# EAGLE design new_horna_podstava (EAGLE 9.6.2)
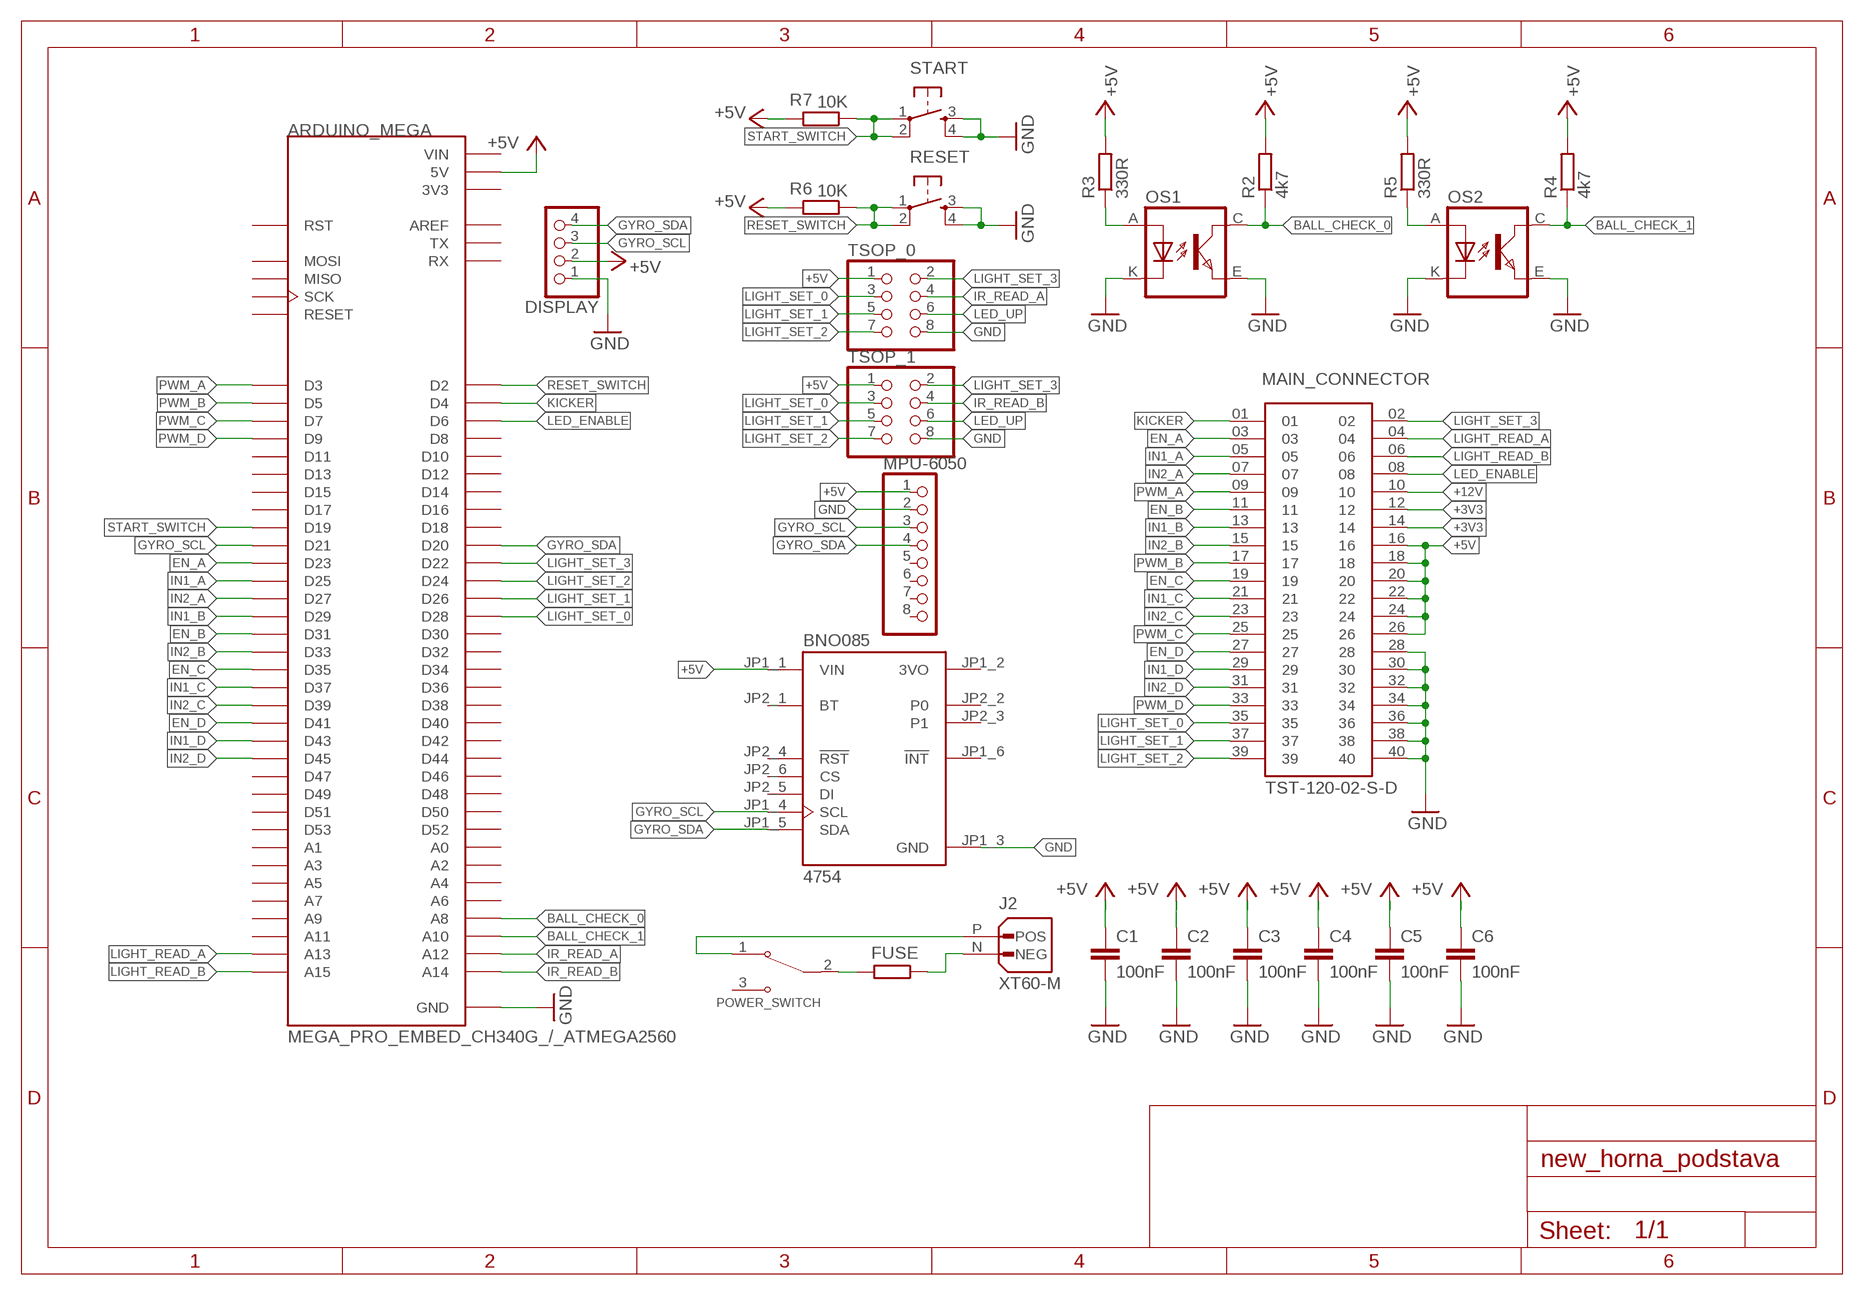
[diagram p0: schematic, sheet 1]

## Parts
ARDUINO_MEGA  MEGA_PRO_EMBED_CH340G_/_ATMEGA2560  [MODULE_MEGA_PRO_EMBED_CH340G_/_ATMEGA2560]
BNO085  4754  [MODULE_4754]
C1  100nF  C-EUC0805  [C0805]
C2  100nF  C-EUC0805  [C0805]
C3  100nF  C-EUC0805  [C0805]
C4  100nF  C-EUC0805  [C0805]
C5  100nF  C-EUC0805  [C0805]
C6  100nF  C-EUC0805  [C0805]
DISPLAY  PINHD-1X4  [1X04]
FUSE  R-EU_R1206  [R1206]
J2  XT60-M  [AMASS_XT60-M]
MAIN_CONNECTOR  TST-120-02-S-D  [SAMTEC_TST-120-02-S-D]
MPU-6050  PINHD-1X8  [1X08]
OS1  TCRT5000  [TCRT5000]
OS2  TCRT5000  [TCRT5000]
POWER_SWITCH  100SP1T1B4M2QE  [SW_100SP1T1B4M2QE]
R2  4k7  R-EU_R1206  [R1206]
R3  330R  R-EU_R1206  [R1206]
R4  4k7  R-EU_R1206  [R1206]
R5  330R  R-EU_R1206  [R1206]
R6  10K  R-EU_R1206  [R1206]
R7  10K  R-EU_R1206  [R1206]
RESET  DTSM-6  [DTSM-6]
START  DTSM-6  [DTSM-6]
TSOP_0  PINHD-2X4  [2X04]
TSOP_1  PINHD-2X4  [2X04]

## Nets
+3V3: MAIN_CONNECTOR.12 MAIN_CONNECTOR.14
+5V: ARDUINO_MEGA.5V_1(5V) ARDUINO_MEGA.5V_2(5V) ARDUINO_MEGA.5V_3(5V) BNO085.JP1_1(VIN) C1.1 C2.1 C3.1 C4.1 C5.1 C6.1 DISPLAY.2 MAIN_CONNECTOR.16 MAIN_CONNECTOR.18 MAIN_CONNECTOR.20 MAIN_CONNECTOR.22 MAIN_CONNECTOR.24 MAIN_CONNECTOR.26 MPU-6050.1 R2.2 R3.2 R4.2 R5.2 R6.2 R7.2 TSOP_0.1 TSOP_1.1
+12V: MAIN_CONNECTOR.10
BALL_CHECK_0: ARDUINO_MEGA.A8 OS1.C(COLLECTOR) R2.1
BALL_CHECK_1: ARDUINO_MEGA.A10 OS2.C(COLLECTOR) R4.1
EN_A: ARDUINO_MEGA.D23 MAIN_CONNECTOR.03
EN_B: ARDUINO_MEGA.D31 MAIN_CONNECTOR.11
EN_C: ARDUINO_MEGA.D35 MAIN_CONNECTOR.19
EN_D: ARDUINO_MEGA.D41 MAIN_CONNECTOR.27
GND: ARDUINO_MEGA.GND_1(GND) ARDUINO_MEGA.GND_2(GND) ARDUINO_MEGA.GND_3(GND) BNO085.JP1_3(GND) C1.2 C2.2 C3.2 C4.2 C5.2 C6.2 DISPLAY.1 MAIN_CONNECTOR.28 MAIN_CONNECTOR.30 MAIN_CONNECTOR.32 MAIN_CONNECTOR.34 MAIN_CONNECTOR.36 MAIN_CONNECTOR.38 MAIN_CONNECTOR.40 MPU-6050.2 OS1.E(EMITTER) OS1.K(CATHODE) OS2.E(EMITTER) OS2.K(CATHODE) RESET.3 RESET.4 START.3 START.4 TSOP_0.8 TSOP_1.8
GYRO_SCL: ARDUINO_MEGA.D21 BNO085.JP1_4(SCL) DISPLAY.3 MPU-6050.3
GYRO_SDA: ARDUINO_MEGA.D20 BNO085.JP1_5(SDA) DISPLAY.4 MPU-6050.4
IN1_A: ARDUINO_MEGA.D25 MAIN_CONNECTOR.05
IN1_B: ARDUINO_MEGA.D29 MAIN_CONNECTOR.13
IN1_C: ARDUINO_MEGA.D37 MAIN_CONNECTOR.21
IN1_D: ARDUINO_MEGA.D43 MAIN_CONNECTOR.29
IN2_A: ARDUINO_MEGA.D27 MAIN_CONNECTOR.07
IN2_B: ARDUINO_MEGA.D33 MAIN_CONNECTOR.15
IN2_C: ARDUINO_MEGA.D39 MAIN_CONNECTOR.23
IN2_D: ARDUINO_MEGA.D45 MAIN_CONNECTOR.31
IR_READ_A: ARDUINO_MEGA.A12 TSOP_0.4
IR_READ_B: ARDUINO_MEGA.A14 TSOP_1.4
KICKER: ARDUINO_MEGA.D4 MAIN_CONNECTOR.01
LED_ENABLE: ARDUINO_MEGA.D6 MAIN_CONNECTOR.08
LED_UP: TSOP_0.6 TSOP_1.6
LIGHT_READ_A: ARDUINO_MEGA.A13 MAIN_CONNECTOR.04
LIGHT_READ_B: ARDUINO_MEGA.A15 MAIN_CONNECTOR.06
LIGHT_SET_0: ARDUINO_MEGA.D28 MAIN_CONNECTOR.35 TSOP_0.3 TSOP_1.3
LIGHT_SET_1: ARDUINO_MEGA.D26 MAIN_CONNECTOR.37 TSOP_0.5 TSOP_1.5
LIGHT_SET_2: ARDUINO_MEGA.D24 MAIN_CONNECTOR.39 TSOP_0.7 TSOP_1.7
LIGHT_SET_3: ARDUINO_MEGA.D22 MAIN_CONNECTOR.02 TSOP_0.2 TSOP_1.2
N$1: FUSE.2 POWER_SWITCH.2
N$2: J2.P(POS) POWER_SWITCH.1
N$3: FUSE.1 J2.N(NEG)
N$5: OS2.A(ANODE) R5.1
N$6: OS1.A(ANODE) R3.1
PWM_A: ARDUINO_MEGA.D3 MAIN_CONNECTOR.09
PWM_B: ARDUINO_MEGA.D5 MAIN_CONNECTOR.17
PWM_C: ARDUINO_MEGA.D7 MAIN_CONNECTOR.25
PWM_D: ARDUINO_MEGA.D9 MAIN_CONNECTOR.33
RESET_SWITCH: ARDUINO_MEGA.D2 R6.1 RESET.1 RESET.2
START_SWITCH: ARDUINO_MEGA.D19 R7.1 START.1 START.2
Unconnected: ARDUINO_MEGA.A0 ARDUINO_MEGA.A1 ARDUINO_MEGA.A2 ARDUINO_MEGA.A3 ARDUINO_MEGA.A4 ARDUINO_MEGA.A5 ARDUINO_MEGA.A6 ARDUINO_MEGA.A7 ARDUINO_MEGA.A9 ARDUINO_MEGA.A11 ARDUINO_MEGA.AREF ARDUINO_MEGA.D8 ARDUINO_MEGA.D10 ARDUINO_MEGA.D11 ARDUINO_MEGA.D12 ARDUINO_MEGA.D13 ARDUINO_MEGA.D14 ARDUINO_MEGA.D15 ARDUINO_MEGA.D16 ARDUINO_MEGA.D17 ARDUINO_MEGA.D18 ARDUINO_MEGA.D30 ARDUINO_MEGA.D32 ARDUINO_MEGA.D34 ARDUINO_MEGA.D36 ARDUINO_MEGA.D38 ARDUINO_MEGA.D40 ARDUINO_MEGA.D42 ARDUINO_MEGA.D44 ARDUINO_MEGA.D46 ARDUINO_MEGA.D47 ARDUINO_MEGA.D48 ARDUINO_MEGA.D49 ARDUINO_MEGA.D50 ARDUINO_MEGA.D51 ARDUINO_MEGA.D52 ARDUINO_MEGA.D53 ARDUINO_MEGA.MISO ARDUINO_MEGA.MOSI ARDUINO_MEGA.RESET ARDUINO_MEGA.RST ARDUINO_MEGA.RX ARDUINO_MEGA.SCK ARDUINO_MEGA.TX ARDUINO_MEGA.VIN_1(VIN) ARDUINO_MEGA.VIN_2(VIN) BNO085.JP1_2(3VO) BNO085.JP1_6(!INT) BNO085.JP2_1(BT) BNO085.JP2_2(P0) BNO085.JP2_3(P1) BNO085.JP2_4(!RST) BNO085.JP2_5(DI) BNO085.JP2_6(CS) MPU-6050.5 MPU-6050.6 MPU-6050.7 MPU-6050.8 POWER_SWITCH.3

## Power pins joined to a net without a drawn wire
3V3: ARDUINO_MEGA.3V3_1(3V3) ARDUINO_MEGA.3V3_2(3V3)

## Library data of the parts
ARDUINO_MEGA = MEGA_PRO_EMBED_CH340G___ATMEGA2560:MEGA_PRO_EMBED_CH340G_/_ATMEGA2560: Mega 2560 PRO (Embed) CH340G/ATmega2560-16AU Check availability; AVAILABILITY: Not in stock; MF: Robotdyn; MP: Mega Pro Embed CH340G / ATmega2560; PACKAGE: None; PRICE: None
BNO085 = 4754:4754: Check availability; AVAILABILITY: In Stock; DESCRIPTION: Adafruit 9-DOF Orientation IMU Fusion Breakout - BNO085 (BNO080) - STEMMA QT / Qwiic; MF: Adafruit; MP: 4754; PACKAGE: None; PRICE: None; PURCHASE-URL: https://pricing.snapeda.com/search/part/4754/?ref=eda
C1-C6 = rcl:C-EU: CAPACITOR, European symbol; SPICEPREFIX: C
DISPLAY = pinhead:PINHD-1X4: PIN HEADER
FUSE R2-R7 = rcl:R-EU_: RESISTOR, European symbol; SPICEPREFIX: R
J2 = XT60-M:XT60-M: Check availability; AVAILABILITY: Not in stock; DESCRIPTION: Plug; DC supply; XT60; male; PIN: 2; for cable; soldered; 30A; 500V; MF: AMASS; MP: XT60-M; PACKAGE: Package; PRICE: None
MAIN_CONNECTOR = TST-120-02-S-D:TST-120-02-S-D: Check availability; AVAILABILITY: In Stock; DESCRIPTION: Connector Header Through Hole 40 position 0.100 (2.54mm); MF: Samtec; MP: TST-120-02-S-D-20; PACKAGE: None; PRICE: None; PURCHASE-URL: https://pricing.snapeda.com/search/part/TST-120-02-S-D-20/?ref=eda
MPU-6050 = pinhead:PINHD-1X8: PIN HEADER
OS1 OS2 = tcrt5000:TCRT5000
POWER_SWITCH = 100SP1T1B4M2QE:100SP1T1B4M2QE: Toggle Switch SPDT Through Hole Check availability; AVAILABILITY: In Stock; DESCRIPTION: Toggle Switch SPDT Through Hole; MF: E-Switch; MP: 100SP1T1B4M2QE; PACKAGE: None; PRICE: None; PURCHASE-URL: https://pricing.snapeda.com/search/part/100SP1T1B4M2QE/?ref=eda
RESET START = switch-tact:DTSM-6
TSOP_0 TSOP_1 = pinhead:PINHD-2X4: PIN HEADER

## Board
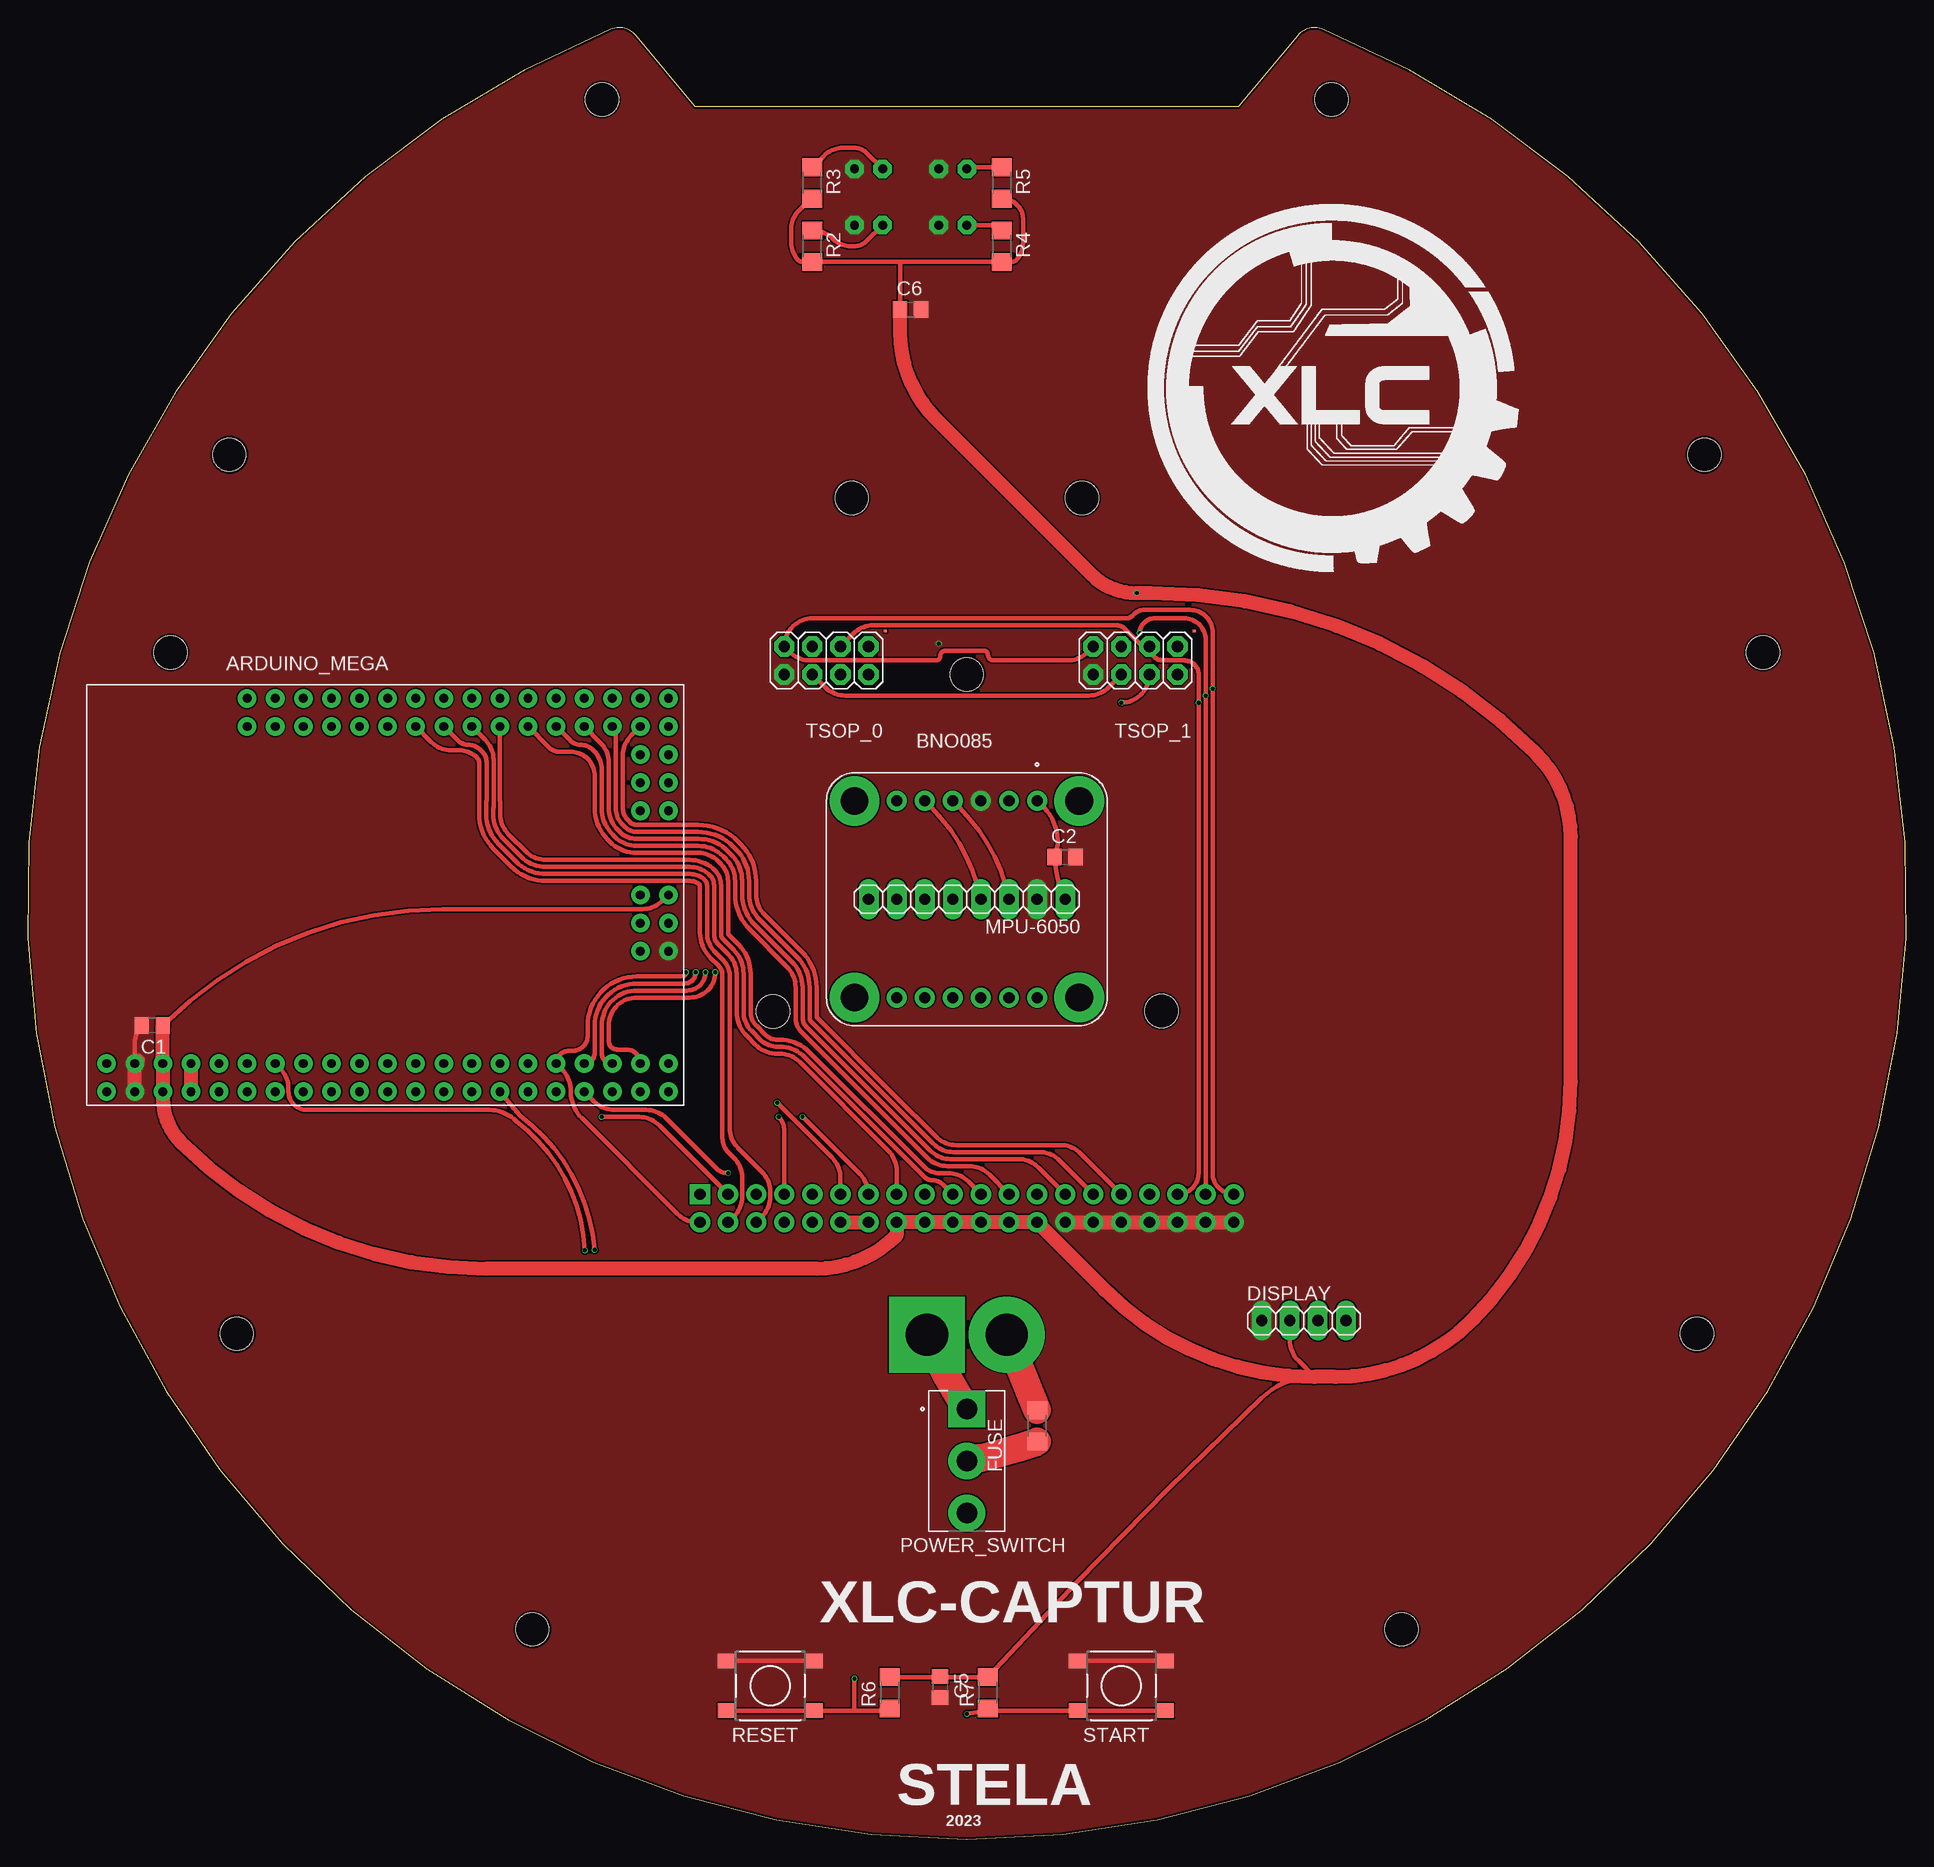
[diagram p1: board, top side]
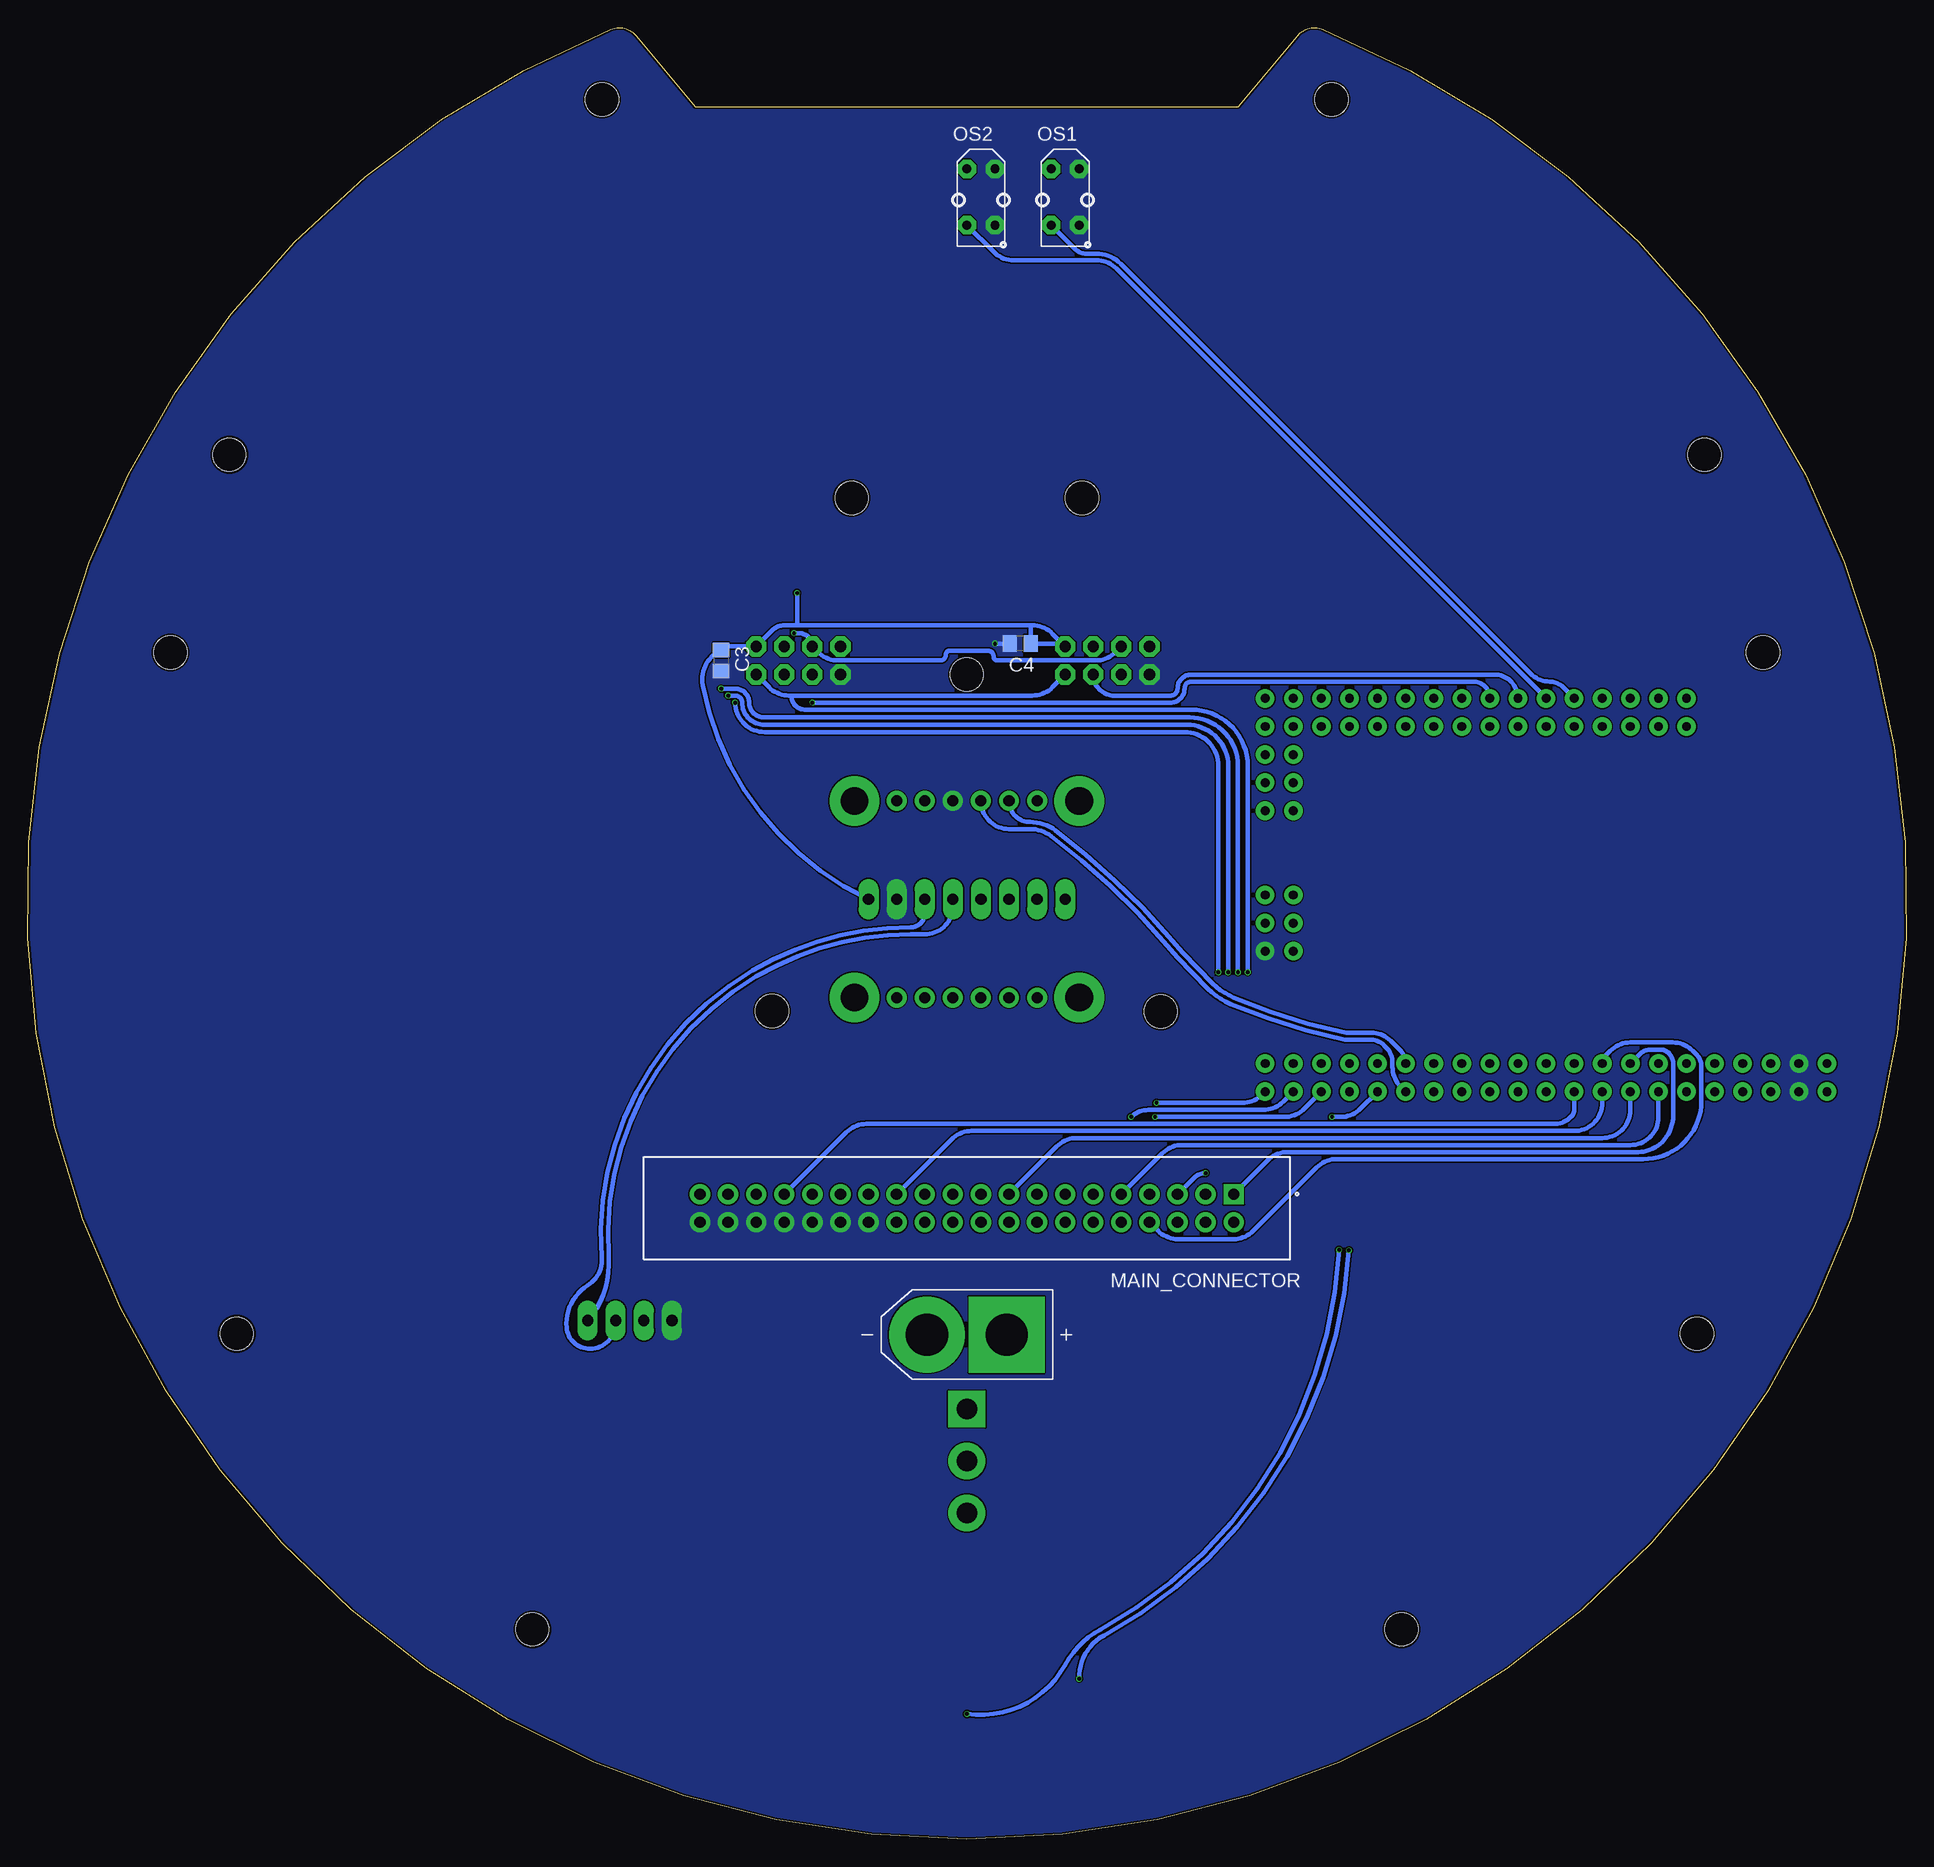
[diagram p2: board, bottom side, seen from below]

Size 169.86 x 163.81 mm. Coordinates in mm from the lower left corner, seen from the top.
Outline: 60.37,156.65 55.03,163.09 arc73 52.73,163.67 arc315 117.13,163.67 arc73 114.83,163.09 109.48,156.65 60.37,156.65
Copper layers (1*16): Top 0.035mm / dielectric 1.6mm / Bottom 0.035mm
Design rules "jlc_pcb": minimum track width 5mil, minimum drill 0.3mm, track to track 5mil, track to pad 5mil, pad to pad 5mil, via to via 5mil, smd to smd 5mil, copper to edge 0.2mm, drill to drill 6mil, minimum pad ring 10mil, minimum via ring 3mil, stop-mask expansion 4mil, vias tented up to drill 0mil, thermal gap 10mil
Holes 3 mm at 156.93,107.32 12.93,107.32 102.54,74.9 67.39,74.86 84.93,105.32 151.62,125.19 150.94,45.71 124.22,18.98 95.34,121.27 74.51,121.27 45.64,18.98 18.91,45.71 18.24,125.19 117.91,157.32 51.94,157.32

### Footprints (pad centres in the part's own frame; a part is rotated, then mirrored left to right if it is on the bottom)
MODULE_MEGA_PRO_EMBED_CH340G_/_ATMEGA2560 = drill 0.8 pad 1.676: 3V3_1 -17.58,-17.78; 3V3_2 -17.58,-15.24; 5V_1 -20.12,-17.78; 5V_2 -20.12,-15.24; 5V_3 25.6,0; A0 -12.5,17.78; A1 -12.5,15.24; A2 -9.96,17.78; A3 -9.96,15.24; A4 -7.42,17.78; A5 -7.42,15.24; A6 -4.88,17.78; A7 -4.88,15.24; A8 -2.34,17.78; A9 -2.34,15.24; A10 0.2,17.78; A11 0.2,15.24; A12 2.74,17.78; A13 2.74,15.24; A14 5.28,17.78; A15 5.28,15.24; AREF -15.04,-15.24; D2 -9.96,-15.24; D3 -9.96,-17.78; D4 -7.42,-15.24; D5 -7.42,-17.78; D6 -4.88,-15.24; D7 -4.88,-17.78; D8 -2.34,-15.24; D9 -2.34,-17.78; D10 0.2,-15.24; D11 0.2,-17.78; D12 2.74,-15.24; D13 2.74,-17.78; D14 5.28,-15.24; D15 5.28,-17.78; D16 7.82,-15.24; D17 7.82,-17.78; D18 10.36,-15.24; D19 10.36,-17.78; D20 12.9,-15.24; D21 12.9,-17.78; D22 15.44,-15.24; D23 15.44,-17.78; D24 17.98,-15.24; D25 17.98,-17.78; D26 20.52,-15.24; D27 20.52,-17.78; D28 23.06,-15.24; D29 23.06,-17.78; D30 25.6,-15.24; D31 25.6,-17.78; D32 7.82,17.78; D33 7.82,15.24; D34 10.36,17.78; D35 10.36,15.24; D36 12.9,17.78; D37 12.9,15.24; D38 15.44,17.78; D39 15.44,15.24; D40 17.98,17.78; D41 17.98,15.24; D42 20.52,17.78; D43 20.52,15.24; D44 23.06,17.78; D45 23.06,15.24; D46 25.6,17.78; D47 25.6,15.24; D48 25.6,12.7; D49 23.06,12.7; D50 25.6,10.16; D51 23.06,10.16; D52 25.6,7.62; D53 23.06,7.62; GND_1 -22.66,-17.78; GND_2 -22.66,-15.24; GND_3 25.6,-5.08; MISO 23.06,0; MOSI 25.6,-2.54; RESET 23.06,-5.08; RST -15.04,-17.78; RX -12.5,-15.24; SCK 23.06,-2.54; TX -12.5,-17.78; VIN_1 -25.2,-17.78; VIN_2 -25.2,-15.24
MODULE_4754 = drill 1 pad 1.778: JP1_1 -6.35,-8.89; JP1_2 -3.81,-8.89; JP1_3 -1.27,-8.89; JP1_4 1.27,-8.89; JP1_5 3.81,-8.89; JP1_6 6.35,-8.89; JP2_1 -6.35,8.89; JP2_2 -3.81,8.89; JP2_3 -1.27,8.89; JP2_4 1.27,8.89; JP2_5 3.81,8.89; JP2_6 6.35,8.89 | drill 2.5 pad 3.2: P1 -10.16,8.89; P2 10.16,8.89; P3 -10.16,-8.89; P4 10.16,-8.89
C0805 = smd 1.3 x 1.5: 1 -0.95,0; 2 0.95,0
1X04 = drill 1.016 long: 1 -3.81,0; 2 -1.27,0; 3 1.27,0; 4 3.81,0
R1206 = smd 1.6 x 1.803: 1 -1.422,0; 2 1.422,0
AMASS_XT60-M = drill 3.81 pad 5.08: N 3.6,0 | drill 3.81 pad 5.08 square: P -3.6,0
SAMTEC_TST-120-02-S-D = drill 1.02 pad 1.37 square: 01 0,0 | drill 1.02 pad 1.37: 02 0,2.54; 03 2.54,0; 04 2.54,2.54; 05 5.08,0; 06 5.08,2.54; 07 7.62,0; 08 7.62,2.54; 09 10.16,0; 10 10.16,2.54; 11 12.7,0; 12 12.7,2.54; 13 15.24,0; 14 15.24,2.54; 15 17.78,0; 16 17.78,2.54; 17 20.32,0; 18 20.32,2.54; 19 22.86,0; 20 22.86,2.54; 21 25.4,0; 22 25.4,2.54; 23 27.94,0; 24 27.94,2.54; 25 30.48,0; 26 30.48,2.54; 27 33.02,0; 28 33.02,2.54; 29 35.56,0; 30 35.56,2.54; 31 38.1,0; 32 38.1,2.54; 33 40.64,0; 34 40.64,2.54; 35 43.18,0; 36 43.18,2.54; 37 45.72,0; 38 45.72,2.54; 39 48.26,0; 40 48.26,2.54
1X08 = drill 1.016 long: 1 -8.89,0; 2 -6.35,0; 3 -3.81,0; 4 -1.27,0; 5 1.27,0; 6 3.81,0; 7 6.35,0; 8 8.89,0
TCRT5000 = drill 0.8 pad 1.676 octagon: A -2.54,-1.27; C 2.54,-1.27; E 2.54,1.27; K -2.54,1.27
SW_100SP1T1B4M2QE = drill 1.85 square: 1 0,4.7 | drill 1.85: 2 0,0; 3 0,-4.7
DTSM-6 = smd 1.55 x 1.3: 1 -3.975,2.25; 2 3.975,2.25; 3 -3.975,-2.25; 4 3.975,-2.25
2X04 = drill 1.016 octagon: 1 -3.81,-1.27; 2 -3.81,1.27; 3 -1.27,-1.27; 4 -1.27,1.27; 5 1.27,-1.27; 6 1.27,1.27; 7 3.81,-1.27; 8 3.81,1.27 | smd 0.254 x 0.254: P$1 -5.334,-2.667

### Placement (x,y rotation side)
ARDUINO_MEGA  32.35,85.38 0 top
BNO085  84.93,85 180 top
C1  11.27,73.57 180 top
C2  93.82,88.81 0 top
C3  107.15,106.59 270 bottom
C4  80.1,108.11 180 bottom
C5  82.51,13.75 270 top
C6  79.85,138.34 0 top
DISPLAY  115.41,46.9 0 top
FUSE  91.28,37.38 270 top
J2  84.93,45.63 180 bottom
MAIN_CONNECTOR  60.8,58.33 180 bottom
MPU-6050  84.93,85 180 top
OS1  76.04,148.5 270 bottom
OS2  83.66,148.5 270 bottom
POWER_SWITCH  84.93,34.2 0 top
R2  70.96,144.06 270 top
R3  70.96,149.77 270 top
R4  88.1,144.06 270 top
R5  88.1,149.77 270 top
R6  77.94,13.25 90 top
R7  86.83,13.25 90 top
RESET  67.15,13.88 180 top
START  98.9,13.88 180 top
TSOP_0  72.23,106.59 180 top
TSOP_1  100.17,106.59 180 top

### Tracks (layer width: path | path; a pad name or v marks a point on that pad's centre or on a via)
3V3
  Top 1.27: ARDUINO_MEGA.3V3_2 ARDUINO_MEGA.3V3_1
+3V3
  Top 1.27: MAIN_CONNECTOR.12 MAIN_CONNECTOR.14
+5V  (via drill 0.35)
  Top 0.406: 78.96,142.63 R4.2 89.01,142.63 arc45 89.37,142.79 arc45 90.01,144.32 90.01,146.6 arc45 89.56,147.68 89.37,147.87 arc45 88.21,148.35 R5.2 | R3.2 arc45 70.7,148.24 69.69,147.23 arc45 69.05,145.7 69.05,144.32 arc45 69.69,142.79 arc45 70.05,142.63 R2.2 71.59,142.63 78.96,142.63 | C6.1 78.9,142.49 arc-45 78.96,142.63 | ARDUINO_MEGA.5V_3 57.42,84.86 arc-45 55.63,84.11 37.49,84.11 arc45 12.41,73.72 12.23,73.54 | DISPLAY.2 114.14,45.09 arc45 114.88,43.29 116.36,41.82 arc44 111.6,39.92 arc4 R7.2 82.39,14.67 | R6.2 82.39,14.67 | C5.1 82.39,14.67 | BNO085.JP1_1 91.91,93.26 arc-66 C2.1 92.93,88.18 arc20 MPU-6050.1
  Top 1.27: C6.1 78.9,136.36 arc45 82.21,128.36 96.19,114.38 arc45 v100.27,112.69 101.52,112.69 arc-45 136.28,98.29 136.45,98.13 arc-45 139.54,90.66 139.54,68.5 arc-45 130.6,46.93 arc-45 118.26,41.82 116.36,41.82 arc-45 97.39,49.68 MAIN_CONNECTOR.26 MAIN_CONNECTOR.24 MAIN_CONNECTOR.22 MAIN_CONNECTOR.20 MAIN_CONNECTOR.18 MAIN_CONNECTOR.16 78.58,54.62 arc-45 71.29,51.6 41.47,51.6 arc-45 13.84,63.05 arc-45 12.23,66.94 ARDUINO_MEGA.5V_1 ARDUINO_MEGA.5V_2 12.23,73.54 arc45 C1.1
  Bottom 0.406: 79.21,109.77 78.99,109.77 arc45 77.2,109.02 TSOP_0.1 arc-45 76.65,108.11 C4.1 79.15,109.62 arc-45 79.21,109.77 | 79.21,109.77 100.27,109.77 | 100.27,109.77 101.45,109.77 arc-45 102.51,109.33 TSOP_1.1 106.38,107.86 arc-45 C3.1 107.64,107.21 arc-66 108.81,104.36 arc-54 MPU-6050.1 | v100.27,112.69 100.27,109.77
BALL_CHECK_0
  Top 0.406: R2.1 71.02,145.48 arc-45 72.82,144.73 72.86,144.69 arc45 74.4,144.06 74.77,144.06 arc45 75.85,144.5 OS1.C
  Bottom 0.406: ARDUINO_MEGA.A8 31.05,104.2 arc-45 32.22,104.69 arc45 33.96,105.4 71.02,142.46 arc-45 73.24,143.38 74.13,143.38 arc45 75.15,143.81 OS1.C
BALL_CHECK_1
  Top 0.406: OS2.C 86.94,145.96 arc-45 R4.1
  Bottom 0.406: ARDUINO_MEGA.A10 71.43,142.04 arc-45 73.23,142.79 80.7,142.79 arc45 82.5,143.53 OS2.C
EN_A  (via drill 0.35)
  Top 0.406: v51.91,65.32 55.3,65.32 arc-45 57.1,64.57 MAIN_CONNECTOR.03
  Bottom 0.406: ARDUINO_MEGA.D23 49.33,66.06 arc45 51.13,65.32 v51.91,65.32
EN_B  (via drill 0.35)
  Top 0.406: v67.78,66.59 72.75,61.61 arc-45 73.5,59.82 MAIN_CONNECTOR.11
  Bottom 0.406: ARDUINO_MEGA.D31 58.22,67.33 arc45 60.02,66.59 v67.78,66.59
EN_C
  Top 0.406: ARDUINO_MEGA.D35 42.71,93.89 42.74,93.86 42.74,92.68 arc45 43.48,90.89 45.07,89.3 arc45 46.86,88.56 59.88,88.56 arc-45 62.14,87.62 arc-45 62.7,86.27 62.7,81.83 | 62.7,81.83 arc45 62.7,81.83 | 62.7,81.83 arc45 62.89,81.38 63.84,80.42 arc-45 64.73,78.27 64.73,74.84 arc45 65.46,73.09 66.25,72.3 arc45 67.78,71.67 68,71.67 arc-45 70.25,70.74 81.12,59.86 arc45 81.75,59.6 arc-45 82.84,59.15 MAIN_CONNECTOR.19
EN_D
  Top 0.406: ARDUINO_MEGA.D41 51.8,99.15 arc-45 52.54,97.36 52.54,93.26 arc45 53.36,91.27 53.55,91.09 arc45 55.06,90.46 60.63,90.46 arc-45 63.33,89.35 63.6,89.07 arc-45 64.61,86.64 64.61,85.42 arc45 65.72,82.72 69.14,79.31 arc-45 70.07,77.06 70.07,74.33 arc45 70.44,73.43 81.63,62.25 arc45 83.42,61.51 89.59,61.51 arc-45 91.39,60.76 MAIN_CONNECTOR.27
GND  (via drill 0.35)
  Top 0.406: ARDUINO_MEGA.GND_2 9.97,70.42 | ARDUINO_MEGA.GND_2 ARDUINO_MEGA.GND_1 | ARDUINO_MEGA.GND_2 9.69,72.05 arc-45 C1.2 | RESET.4 RESET.3 | START.4 START.3
  Top 1.27: MAIN_CONNECTOR.28 MAIN_CONNECTOR.30 MAIN_CONNECTOR.32 MAIN_CONNECTOR.34 MAIN_CONNECTOR.36 MAIN_CONNECTOR.38 MAIN_CONNECTOR.40 | ARDUINO_MEGA.GND_1 9.69,69.74 arc-45 9.97,70.42
  Bottom 0.406: C4.2 v82.39,108.11
  pour Bottom (no thermals): -11.59,168.82 -11.59,-19.77 154.78,-19.77 188.43,-19.77 188.43,145.33 188.43,168.82
  pour Top (no thermals): -11.59,168.82 -11.59,-19.77 188.43,-19.77 188.43,168.82
GYRO_SCL
  Top 0.406: BNO085.JP1_4 84.29,93.26 arc-33 MPU-6050.3
  Bottom 0.406: ARDUINO_MEGA.D21 45.7,68.05 arc45 46.45,69.85 46.45,70.27 arc-45 46.99,71.57 47.18,71.76 arc-45 48.48,72.3 arc1 50.76,72.31 arc12 61.05,75.53 arc21 63.15,76.93 arc5 67.15,81.19 arc-13 77.31,90.72 arc-37 79.21,91.35 81.12,91.35 arc90 BNO085.JP1_4 | MPU-6050.3 88.74,83.73 arc90 90.01,82.46 arc-31 104.3,78.56 arc-64 117.95,52.57 arc62 119.22,50.08 arc-63 121.12,46.27 arc-80 119.22,44.36 arc-100 DISPLAY.3
GYRO_SDA
  Top 0.406: BNO085.JP1_5 81.75,93.26 arc-33 MPU-6050.4
  Bottom 0.406: ARDUINO_MEGA.D20 arc-45 45.75,71.35 46.62,72.22 arc-45 48.35,72.94 50.64,72.94 arc12 60.8,76.11 arc21 62.7,77.38 arc5 66.67,81.6 arc-13 76.93,91.22 arc-37 79.21,91.99 arc90 BNO085.JP1_5 | MPU-6050.4 86.2,84.37 arc90 88.74,81.83 90.01,81.83 arc-31 103.98,78.02 arc-64 117.31,52.62 arc45 DISPLAY.4
IN1_A  (via drill 0.35)
  Top 0.406: ARDUINO_MEGA.D25 51.24,66.69 arc45 53.03,65.95 55.94,65.95 arc-45 57.73,65.21 62.25,60.68 arc45 v63.34,60.24
  Bottom 0.406: v63.34,60.24 arc-45 64.42,59.79 MAIN_CONNECTOR.05
IN1_B  (via drill 0.35)
  Top 0.406: MAIN_CONNECTOR.13 arc45 75.32,60.06 v70.07,65.32
  Bottom 0.406: ARDUINO_MEGA.D29 56.32,66.69 arc45 58.11,65.95 68.54,65.95 arc-45 v70.07,65.32
IN1_C
  Top 0.406: ARDUINO_MEGA.D37 47.14,98.73 arc45 48.1,98.34 49.1,98.34 arc-45 50.64,97.7 arc-45 51.27,96.17 51.27,93.26 arc45 52.47,90.38 52.65,90.19 arc45 55.06,89.19 60.63,89.19 arc-45 62.43,88.45 62.7,88.18 arc-45 63.34,86.64 63.34,84.15 | 63.34,84.15 arc-45 63.34,84.15 | 63.34,84.15 63.34,81.83 64.29,80.87 arc-45 65.37,78.27 65.37,74.84 arc45 65.91,73.54 66.7,72.75 arc45 67.78,72.3 68,72.3 arc-45 70.69,71.18 81.12,60.76 arc45 82.39,60.24 83.24,60.24 arc-45 85.04,59.49 MAIN_CONNECTOR.21
IN1_D
  Top 0.406: ARDUINO_MEGA.D43 arc-45 53.18,99.88 53.18,93.26 arc45 53.81,91.72 54,91.54 arc45 55.06,91.1 60.63,91.1 arc-45 63.78,89.79 64.05,89.52 arc-45 65.24,86.64 65.24,85.42 arc45 66.17,83.17 69.59,79.76 arc-45 70.7,77.06 70.7,74.33 arc45 70.89,73.88 81.89,62.88 arc45 83.68,62.14 91.5,62.14 arc-45 93.29,61.4 MAIN_CONNECTOR.29
IN2_A  (via drill 0.35)
  Top 0.406: MAIN_CONNECTOR.07 68.42,64.09 arc45 v67.91,65.32
  Bottom 0.406: ARDUINO_MEGA.D27 54.41,66.06 arc45 56.21,65.32 v67.91,65.32
IN2_B
  Top 0.406: ARDUINO_MEGA.D33 41.38,99.41 arc-45 42.13,97.61 42.13,93.28 42.1,93.26 42.1,92.68 arc45 43.03,90.44 44.62,88.85 arc45 46.86,87.92 59.88,87.92 arc-45 61.7,87.17 arc-45 62.07,86.27 62.07,81.83 | 62.07,81.83 arc45 62.07,81.83 | 62.07,81.83 arc45 62.44,80.93 63.39,79.97 arc-45 64.1,78.27 64.1,74.84 arc45 65.01,72.64 65.8,71.85 arc45 67.78,71.03 68,71.03 arc-45 69.8,70.29 77.83,62.25 arc-45 78.58,60.45 MAIN_CONNECTOR.15
IN2_C
  Top 0.406: ARDUINO_MEGA.D39 49.04,99.37 arc45 50,98.97 arc-45 51.09,98.52 51.27,98.34 arc-45 51.91,96.8 51.91,93.26 arc45 52.91,90.82 53.1,90.64 arc45 55.06,89.83 60.63,89.83 arc-45 62.88,88.9 63.15,88.62 arc-45 63.97,86.64 63.97,85.42 arc45 65.27,82.27 68.69,78.86 arc-45 69.43,77.06 69.43,74.33 arc45 69.99,72.99 81.36,61.61 arc45 83.16,60.87 85.15,60.87 arc-45 86.94,60.13 MAIN_CONNECTOR.23
IN2_D
  Top 0.406: ARDUINO_MEGA.D45 54.56,99.77 arc45 53.81,97.97 53.81,93.26 arc45 54.26,92.17 54.45,91.99 arc45 55.06,91.73 60.63,91.73 arc-45 64.23,90.24 64.5,89.97 arc-45 65.88,86.64 65.88,85.42 arc45 66.62,83.62 70.04,80.21 arc-45 71.34,77.06 71.34,74.33 77.88,67.79 78.2,67.47 82.15,63.52 arc45 83.95,62.78 93.4,62.78 arc-45 95.2,62.03 MAIN_CONNECTOR.31
IR_READ_A
  Bottom 0.406: ARDUINO_MEGA.A12 arc-90 37.25,105.32 64.61,105.32 arc-90 65.88,104.05 arc90 66.51,103.42 69.05,103.42 71.59,103.42 arc90 TSOP_0.4
IR_READ_B  (via drill 0.35)
  Top 0.406: TSOP_1.4 arc-90 v98.9,102.78
  Bottom 0.406: ARDUINO_MEGA.A14 arc-90 39.15,104.69 64.61,104.69 arc-90 65.24,104.05 arc90 66.51,102.78 v98.9,102.78
KICKER
  Bottom 0.406: MAIN_CONNECTOR.01 57.73,61.4 arc45 55.94,62.14 24.23,62.14 arc-45 22.06,63.04 arc-45 21.05,65.48 21.05,70.06 arc-45 21.48,71.1 arc-45 22.22,71.41 23.08,71.41 arc-45 24.07,71 ARDUINO_MEGA.D4
LED_ENABLE
  Bottom 0.406: MAIN_CONNECTOR.08 67.64,55.01 arc-45 65.84,54.27 60.8,54.27 arc-45 59.06,54.98 53.29,60.76 arc45 51.49,61.51 23.75,61.51 arc-45 20.04,63.04 arc-45 18.51,66.75 18.51,69.89 arc-45 18.96,70.97 19.29,71.3 arc-45 21.08,72.05 24.95,72.05 arc-45 26.74,71.3 27.16,70.88 arc-45 ARDUINO_MEGA.D6
LED_UP
  Top 0.406: TSOP_0.6 72.12,104.16 arc45 73.91,103.42 95.94,103.42 arc45 97.74,104.16 TSOP_1.6
LIGHT_READ_A
  Top 0.406: ARDUINO_MEGA.A13 36.5,99.21 arc45 38.3,98.46 39.07,98.46 arc-45 40.6,97.83 arc-45 40.86,97.21 40.86,93.89 40.83,93.86 40.83,92.68 arc45 42.13,89.54 43.72,87.95 arc45 46.86,86.65 59.88,86.65 arc-45 60.8,86.27 60.8,81.98 arc45 61.73,79.72 62.49,78.96 arc-45 62.83,78.14 62.83,63.37 arc45 63.34,62.14 63.86,61.61 arc-45 64.61,59.82 64.61,58.11 arc-45 63.86,56.32 MAIN_CONNECTOR.04
LIGHT_READ_B
  Top 0.406: ARDUINO_MEGA.A15 38.88,99.37 arc45 39.84,98.97 arc-45 40.93,98.52 41.11,98.34 arc-45 41.49,97.42 41.49,93.89 41.47,93.86 41.47,92.68 arc45 42.58,89.99 44.17,88.4 arc45 46.86,87.29 59.88,87.29 arc-45 61.25,86.72 arc-45 61.43,86.27 61.43,81.99 arc45 62.18,80.19 62.95,79.42 arc-45 63.48,78.14 63.48,69.13 63.48,68.49 63.48,64.32 arc45 64.22,62.53 66.4,60.34 arc-45 67.15,58.55 67.15,58.11 arc-45 66.4,56.32 MAIN_CONNECTOR.06
LIGHT_SET_0  (via drill 0.35)
  Top 0.406: TSOP_0.3 74.66,109.02 arc-45 76.45,109.77 98.48,109.77 arc-45 99.19,109.47 100.8,107.86 TSOP_1.3 arc90 102.71,106.59 104.61,106.59 arc-90 105.88,105.32 v105.88,102.78 105.88,60.24 arc-90 MAIN_CONNECTOR.35 | ARDUINO_MEGA.D28 arc90 54.14,71.41 53.3,71.41 arc-90 52.54,72.17 52.54,73.57 arc-90 55.08,76.11 59.89,76.11 arc90 v62.18,78.4
  Bottom 0.406: v62.18,78.4 62.18,97.07 arc-90 65.23,100.11 103.22,100.11 arc90 v105.88,102.78
LIGHT_SET_1  (via drill 0.35)
  Top 0.406: MAIN_CONNECTOR.37 v106.52,103.42 106.52,108.5 arc90 104.61,110.4 101.9,110.4 arc90 v100.56,109.06 | ARDUINO_MEGA.D26 arc-90 51.91,71.1 51.91,73.57 arc-90 55.08,76.75 59.64,76.75 arc90 v61.29,78.4
  Bottom 0.406: TSOP_0.5 71.48,107.33 arc45 73.28,106.59 82.13,106.59 arc90 82.51,106.97 arc-90 83.02,107.48 86.45,107.48 arc-90 86.83,107.1 arc90 87.34,106.59 96.58,106.59 arc45 98.37,107.33 TSOP_1.5 arc-90 100.09,109.06 v100.56,109.06 | v61.29,78.4 61.29,97.07 arc-90 65.01,100.78 103.24,100.78 arc90 105.25,102.78 arc-90 105.88,103.42 v106.52,103.42
LIGHT_SET_2  (via drill 0.35)
  Top 0.406: TSOP_1.7 95.83,107.33 arc-45 94.04,106.59 87.34,106.59 arc-90 86.83,107.1 arc90 86.45,107.48 83.02,107.48 arc90 82.51,106.97 arc-90 82.13,106.59 70.74,106.59 arc-45 68.94,107.33 TSOP_0.7 arc-90 70.96,110.4 99.3,110.4 arc45 99.91,110.65 100.06,110.8 arc-45 100.93,111.16 105.12,111.16 arc-90 107.15,109.13 v107.15,104.05 107.15,60.24 arc90 MAIN_CONNECTOR.39 | ARDUINO_MEGA.D24 arc90 51.27,71.08 51.27,73.57 arc-90 55.08,77.38 59.39,77.38 arc90 v60.41,78.4
  Bottom 0.406: v60.41,78.4 60.41,97.07 arc-90 64.79,101.44 103.27,101.44 arc90 104.61,102.78 arc-90 105.88,104.05 v107.15,104.05
LIGHT_SET_3  (via drill 0.35)
  Top 0.406: MAIN_CONNECTOR.02 60.58,55.79 arc-45 58.78,56.53 50.09,65.23 arc-45 49.11,67.59 49.11,67.68 arc45 48.31,69.62 ARDUINO_MEGA.D22 arc-90 48.93,71.28 49.24,71.28 arc90 50.64,72.68 50.64,73.57 arc-90 55.08,78.02 59.15,78.02 arc90 v59.53,78.4
  Bottom 0.406: TSOP_1.2 102.82,104.16 arc-45 101.02,103.42 100.8,103.42 | TSOP_0.2 77.2,104.16 arc45 78.99,103.42 100.8,103.42 | 100.8,103.42 arc-90 99.53,102.15 64.61,102.15 arc90 59.53,97.07 v59.53,78.4
N$1
  Top 2.54: POWER_SWITCH.2 86.07,34.45 arc7 FUSE.2
N$2
  Top 2.54: POWER_SWITCH.1 84.29,39.92 arc-9 J2.P
N$3
  Top 2.54: FUSE.1 J2.N
N$5
  Top 0.406: OS2.A arc-45 85.29,151.19 R5.1
N$6
  Top 0.406: OS1.A 75.85,152.5 arc45 74.77,152.95 73.76,152.95 arc45 71.97,152.2 R3.1
PWM_A
  Bottom 0.406: ARDUINO_MEGA.D3 22.39,65.32 arc90 24.93,62.78 65.46,62.78 arc-45 67.26,62.03 MAIN_CONNECTOR.09
PWM_B
  Bottom 0.406: ARDUINO_MEGA.D5 24.93,65.95 arc90 27.47,63.41 74.99,63.41 arc-45 76.78,62.67 MAIN_CONNECTOR.17
PWM_C
  Bottom 0.406: ARDUINO_MEGA.D7 27.47,66.59 arc90 30.01,64.05 84.51,64.05 arc-45 86.31,63.3 MAIN_CONNECTOR.25
PWM_D
  Bottom 0.406: ARDUINO_MEGA.D9 30.01,65.95 arc45 30.24,65.39 30.32,65.32 arc45 31.85,64.68 94.04,64.68 arc-45 95.83,63.94 MAIN_CONNECTOR.33
RESET_SWITCH  (via drill 0.35)
  Top 0.406: ARDUINO_MEGA.D2 22.84,69.69 arc-45 23.59,67.89 23.59,67.6 arc90 25.24,65.95 41.75,65.95 arc-46 44.16,64.93 arc-50 v50.38,53.25 | RESET.2 RESET.1 74.77,11.63 | 74.77,11.63 77.94,11.63 R6.1 | v74.77,14.52 74.77,11.63
  Bottom 0.406: v50.38,53.25 arc58 72.56,18.4 arc-64 v74.77,14.52
START_SWITCH  (via drill 0.35)
  Top 0.406: ARDUINO_MEGA.D19 44.54,65.44 arc-48 v51.27,53.3 | 86.83,11.63 START.2 START.1 | 86.83,11.63 86.2,11.63 R7.1 | v84.93,11.34 86.83,11.63
  Bottom 0.406: v51.27,53.3 arc58 72.86,18.96 arc-33 76.04,15.79 arc70 v84.93,11.34

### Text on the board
tNames: XLC-CAPTUR | 2023 | STELA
